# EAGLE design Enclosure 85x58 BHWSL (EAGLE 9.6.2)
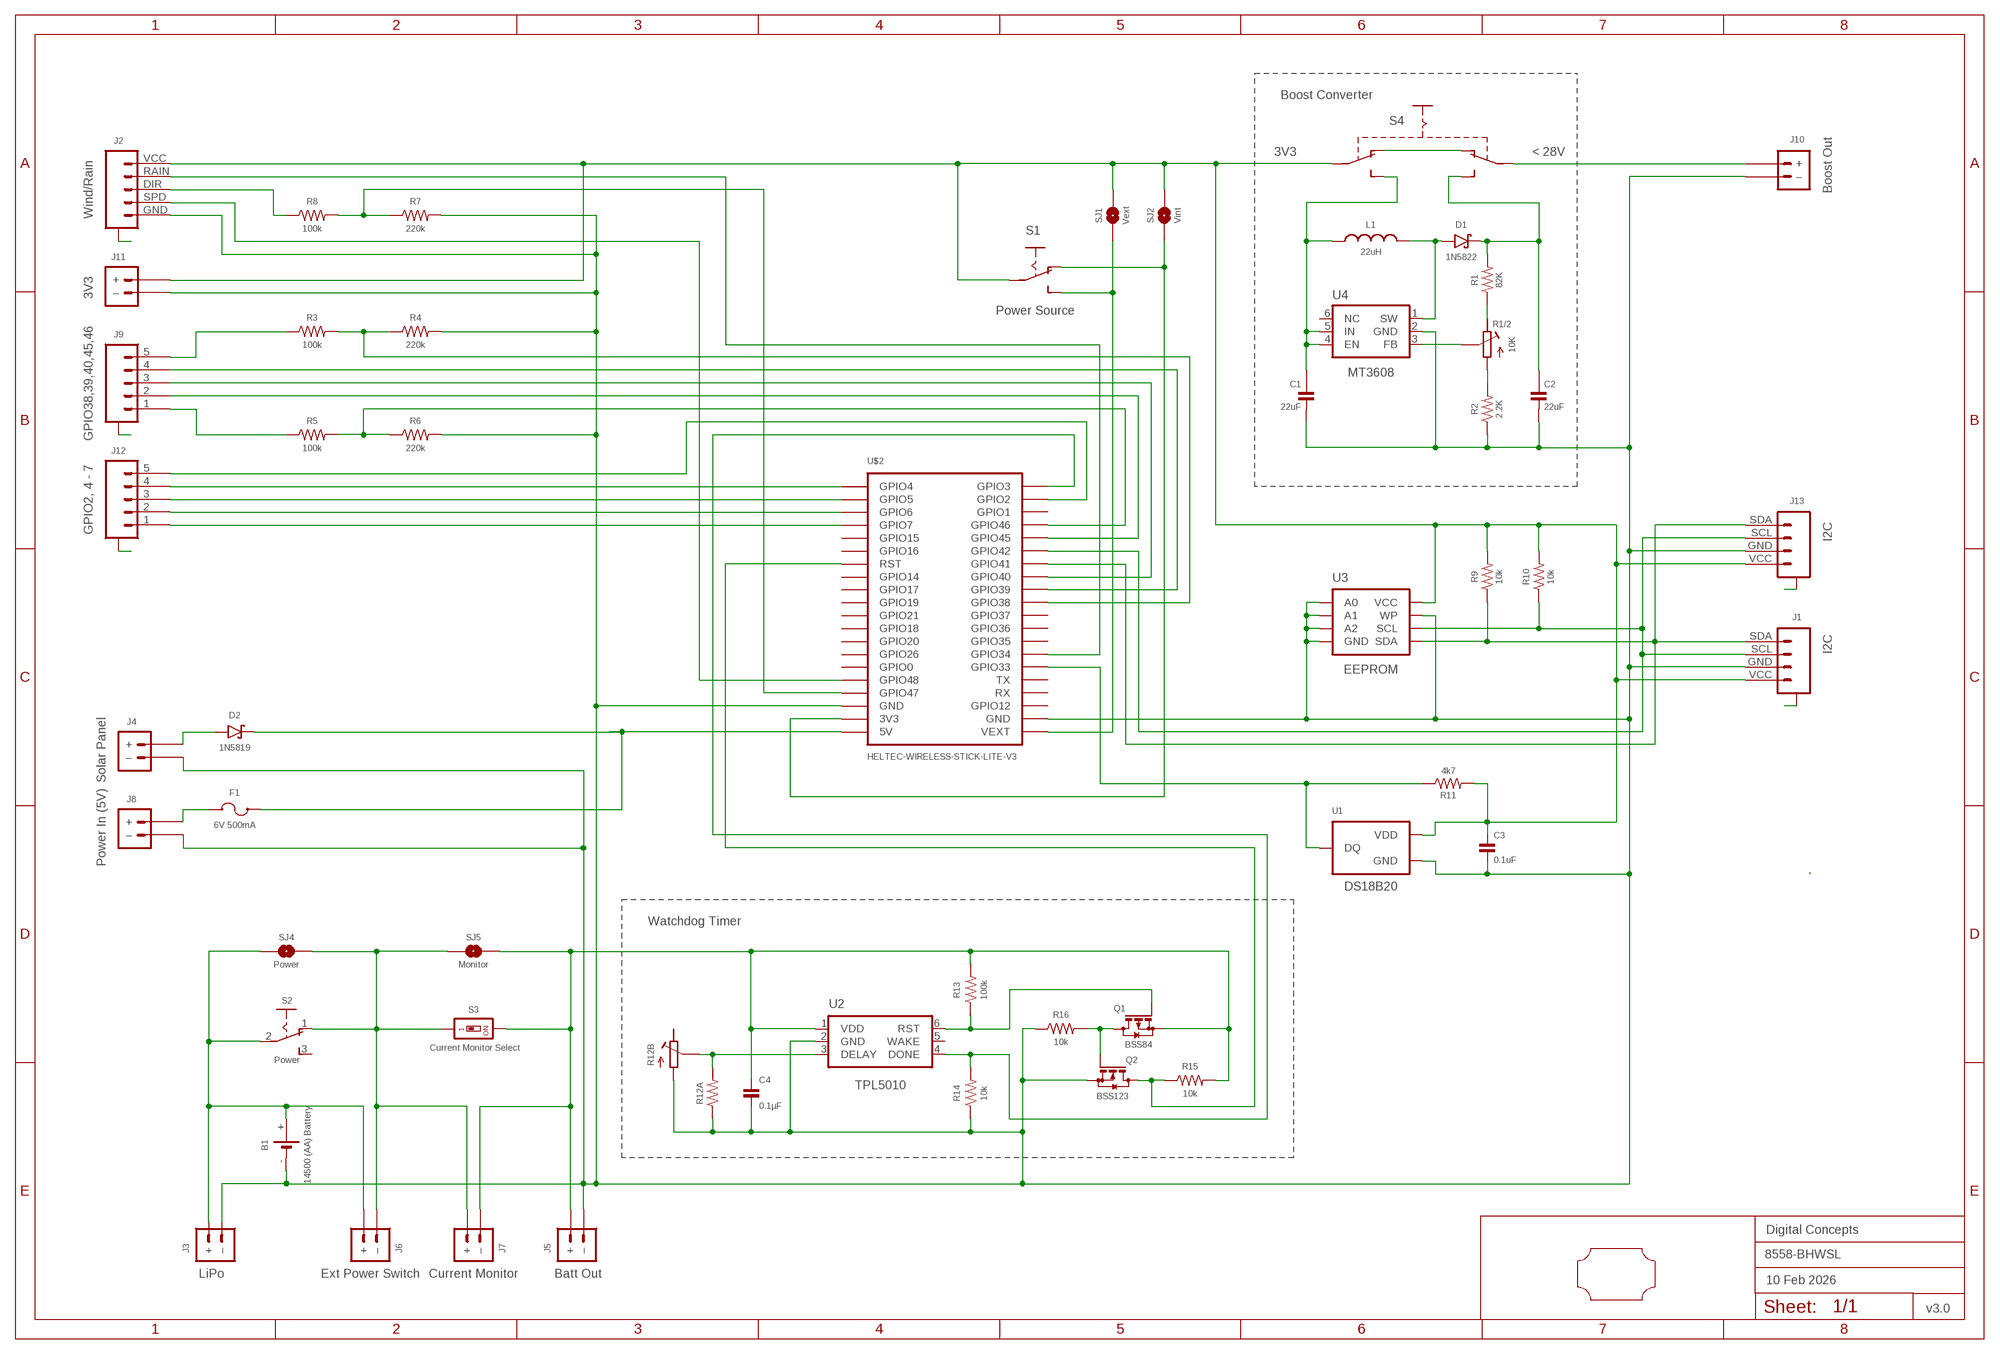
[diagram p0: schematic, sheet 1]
FRAME2 (A3L-LOC): DATE: 10 Feb 2026; OWNER: Digital Concepts; TITLE: 8558-BHWSL; VERSION: v3.0

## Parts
B1  14500 (AA) Battery  BATTERY-HOLDER-14500(AA)  [BATTERY-14500]
C1  22uF  CAPACITOR-1206  [C1206]
C2  22uF  CAPACITOR-1206  [C1206]
C3  0.1uF  CAPACITOR-0805  [C0805]
C4  0.1µF  CAPACITOR-0805  [C0805]
D1  1N5822  DIODE-SCHOTTKY-1N5822  [DIODE_SMB]
D2  1N5819  1N5819-SOD-123  [SOD-123]
F1  6V 500mA  MF-PSMF050X-2  [F0805]
J1  I2C  JST-SH1.0-4-SMD-VERTICAL-I2C  [JST-SH1.0-4-SMD-VERTICAL-I2C]
J2  Wind/Rain  JST-SH1.0-5-SMD-VERTICAL-WEATHER  [JST-SH1.0-5-SMD-VERTICAL-WEATHER]
J3  LiPo  JST-PH2.0-2-MALE-HORIZONTALJST-PTH-2  [JST-PH2.0-2-HORIZONTAL]
J4  Solar Panel  JST-PH2.0-2-VERTICAL-POWER  [JST-PH2.0-2-VERTICAL-POWER]
J5  Batt Out  JST-GH1.25-2-HORIZONTAL-POWER  [JST-GH1.25-2-HORIZONTAL]
J6  Ext Power Switch  JST-PH2.0-2-DUAL-POWERJST-PTH-2  [JST-PH2.0-2-DUAL-POWER]
J7  Current Monitor  JST-PH2.0-2-HORIZONTAL-POWERJST-PTH-2  [JST-PH2.0-2-HORIZONTAL-POWER@1]
J8  Power In (5V)  JST-PH2.0-2-H-POWER  [JST-PH2.0-2-HORIZONTAL-POWER]
J9  GPIO38,39,40,45,46  JST-SH1.0-5-SMD-HORIZONTAL  [JST-SH1.0-5-SMD-HORIZONTAL]
J10  Boost Out  JST-PH2.0-2-H-POWER  [JST-PH2.0-2-HORIZONTAL-POWER]
J11  3V3  JST-PH2.0-2-H-POWER  [JST-PH2.0-2-HORIZONTAL-POWER]
J12  GPIO2, 4 - 7  JST-SH1.0-5-SMD-HORIZONTAL  [JST-SH1.0-5-SMD-HORIZONTAL]
J13  I2C  JST-SH1.0-4-SMD-HORIZONTAL-I2C  [JST-SH1.0-4-SMD-HORIZONTAL-I2C]
L1  22uH  INDUCTOR-CDRH104R/6D28L5038P  [CDRH104R+6D28]
Q1  BSS84  MOSFET-BSS84  [SOT23-3]
Q2  BSS123  MOSFET-BSS123  [SOT23-3]
R1  82K  RESISTORR0805  [R0805]
R1/2  10K  RESISTOR-TRIMM-BAOTER-HORIZONTAL  [RTRIM64P]
R2  2.2K  RESISTORR0805  [R0805]
R3  100k  RESISTORR0805  [R0805]
R4  220k  RESISTORR0805  [R0805]
R5  100k  RESISTORR0805  [R0805]
R6  220k  RESISTORR0805  [R0805]
R7  220k  RESISTORR0805  [R0805]
R8  100k  RESISTORR0805  [R0805]
R9  10k  RESISTORR0805  [R0805]
R10  10k  RESISTORR0805  [R0805]
R11  4k7  RESISTORR0805  [R0805]
R12A  RESISTORR0805  [R0805]
R12B  RESISTOR-TRIMM-33  [RTRIM3*3]
R13  100k  RESISTORR0805  [R0805]
R14  10k  RESISTORR0805  [R0805]
R15  10k  RESISTORR0805  [R0805]
R16  10k  RESISTORR0805  [R0805]
S1  Power Source  SWITCH-SLIDE-SPDT-SMT  [SWITCH-SPDT-SMT]
S2  Power  SWITCH-SLIDE-SPDT  [SWITCH-SLIDE-SPDT]
S3  Current Monitor Select  SWITCH-DIP-SWS001  [SMD-001]
S4  SWITCH-SLIDE-DPDT-PTH-S  [SWITCH-DPDT-PTH]
SJ1  Vext  SJ  [SJ]
SJ2  Vint  SJ-V-1  [SJ-VIA-1]
SJ4  Power  SJ  [SJ]
SJ5  Monitor  SJ  [SJ]
U1  DS18B20  THERMOMETER-DS18B20  [TO-92]
U2  TPL5010  TPL5010DDCR  [SOT-23-6]
U3  EEPROM  AT24CXX-EEPROM  [SOP-8]
U4  MT3608  [SOT-23-6@1]
U$1  PCB-OUTLINE-85X58  [PROTO-28X18-OUTLINE]
U$2  HELTEC-WIRELESS-STICK-LITE-V3  [HELTEC-WIRELESS-STICK-LITE-V3]

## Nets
A1: J1.A@1(A) J1.A@4(A)
A2: J2.A@1(A) J2.A@5(A)
A9: J9.A@1(A) J9.A@5(A)
A12: J12.A@1(A) J12.A@5(A)
A13: J13.A@1(A) J13.A@4(A)
GND: B1.- C1.2 C2.2 C3.2 C4.2 J1.GND J2.GND J3.-(–) J4.-(–) J5.-(–) J8.-(–) J10.-(–) J11.-(–) J13.GND Q2.2(S) R2.1 R4.2 R6.2 R7.2 R12A.1 R12B.1(A) R14.1 R16.1 U1.1(GND) U2.2(GND) U3.P$1(A0) U3.P$2(A1) U3.P$3(A2) U3.P$4(GND) U3.P$7(WP) U4.2(GND) U$2.GND@18(GND) U$2.GND@22(GND)
N$1: D2.A J4.+
N$2: J2.DIR R8.1
N$3: R1.1 R1/2.3(E)
N$4: B1.+ J3.+ J6.+ S2.2(P) SJ4.2
N$5: D2.C F1.2 U$2.5V
N$6: D1.A L1.1 U4.1(SW)
N$7: R7.1 R8.2 U$2.GPIO47
N$8: J1.SCL J13.SCL R10.1 U3.P$6(SCL) U$2.GPIO42
N$9: J9.1 R5.1
N$10: J12.5 U$2.GPIO2
N$11: J1.SDA J13.SDA R9.1 U3.P$5(SDA) U$2.GPIO41
N$12: J2.SPD U$2.GPIO48
N$13: S1.P$1(O) SJ2.2 U$2.3V3
N$14: C4.1 J5.+ J7.-(–) Q1.2(S) R13.2 R15.2 S3.2 SJ5.1 U2.1(VDD)
N$15: J12.4 U$2.GPIO4
N$16: J12.3 U$2.GPIO5
N$18: R11.1 U1.2(DQ) U$2.GPIO33
N$19: J12.2 U$2.GPIO6
N$20: C2.1 D1.C R1.2 S4.P$3(S1)
N$21: S1.P$2(S) SJ1.2 U$2.VEXT
N$22: J2.RAIN U$2.GPIO34
N$23: R1/2.1(A) R2.2
N$24: R1/2.2(S) U4.3(FB)
N$25: C1.1 L1.2 S4.P$6(S2) U4.4(EN) U4.5(IN)
N$26: S4.P$1(O1) S4.P$4(O2)
N$27: J10.+ S4.P$2(P1)
N$28: J12.1 U$2.GPIO7
N$29: J9.2 U$2.GPIO45
N$30: J9.3 U$2.GPIO40
N$31: J9.4 U$2.GPIO39
N$32: J9.5 R3.1
N$33: R3.2 R4.1 U$2.GPIO38
N$34: R5.2 R6.1 U$2.GPIO46
N$35: Q2.3(D) R15.1 U$2.RST
N$38: R14.2 U2.4(DONE) U$2.GPIO3
N$39: J6.-(–) J7.+ S2.1(O) S3.1 SJ4.1 SJ5.2
N$40: F1.1 J8.+
N$43: Q1.3(D) Q2.1(G) R16.2
N$44: Q1.1(G) R13.1 U2.6(RST)
N$46: R12A.2 R12B.2(S) U2.3(DELAY)
VCC: C3.1 J1.VCC J2.VCC J11.+ J13.VCC R9.2 R10.2 R11.2 S1.COMMON(P) S4.P$5(P2) SJ1.1 SJ2.1 SJ2.1@V U1.3(VDD) U3.P$8(VCC)
Unconnected: R12B.3(E) S2.3(S) U2.5(WAKE) U4.6(NC) U$2.GPIO0 U$2.GPIO1 U$2.GPIO12 U$2.GPIO14 U$2.GPIO15 U$2.GPIO16 U$2.GPIO17 U$2.GPIO18 U$2.GPIO19 U$2.GPIO20 U$2.GPIO21 U$2.GPIO26 U$2.GPIO35 U$2.GPIO36 U$2.GPIO37 U$2.RX U$2.TX

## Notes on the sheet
- Boost Converter
- 3V3 | < 28V
- Watchdog Timer

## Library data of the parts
B1 = digitalconcepts:BATTERY-HOLDER-14500(AA): 14500 (AA) battery holder
C1 C2 = digitalconcepts:CAPACITOR-1206: 1206 Capacitor
C3 C4 = digitalconcepts:CAPACITOR-0805: 0805 Capacitor
D1 = digitalconcepts:DIODE-SCHOTTKY-1N5822: 1N5822 Schottky Diode SMB
D2 = digitalconcepts:1N5819-SOD-123: 1N5819 Schottky Diode SOD-123
F1 = digitalconcepts:MF-PSMF050X-2: PTC Resettable Fuse
J1 = digitalconcepts:JST-SH1.0-4-SMD-VERTICAL-I2C: JST SH1.0 4P SMD I2C vertical connector
J2 = digitalconcepts:JST-SH1.0-5-SMD-VERTICAL-WEATHER: JST SH1.0 5P SMD Vertical Weather Connector
J3 = digitalconcepts:JST-PH2.0-2-MALE-HORIZONTAL: PH2.0 2P Right Angle PCB Connector; PROD_ID: CONN-09863; SKU: PRT-09914
J4 = digitalconcepts:JST-PH2.0-2-VERTICAL-POWER: JST PH2.0 2P PTH Connector (Power)
J5 = digitalconcepts:JST-GH1.25-2-HORIZONTAL-POWER: JST GH1.25 2P PTH Connector (Power)
J6 = digitalconcepts:JST-PH2.0-2-DUAL-POWER: JST PH2.0 2P PTH Dual-Side Connector (Power); PROD_ID: CONN-09863; SKU: PRT-09914
J7 = digitalconcepts:JST-PH2.0-2-HORIZONTAL-POWER: PH2.0 2P Right Angle PCB Connector; PROD_ID: CONN-09863; SKU: PRT-09914
J8 J10 J11 = digitalconcepts:JST-PH2.0-2-H-POWER: JST PH2.0 2P Right Angle Connector with power pin labelling
J9 J12 = digitalconcepts:JST-SH1.0-5-SMD-HORIZONTAL: JST SH1.0 5P SMD horizontal connector
J13 = digitalconcepts:JST-SH1.0-4-SMD-HORIZONTAL-I2C: JST SH1.0 4P SMD I2C horizontal connector
L1 = digitalconcepts:INDUCTOR-CDRH104R/6D28: Inductor; SPICEPREFIX: L
Q1 = digitalconcepts:MOSFET-BSS84: P-CHANNEL MOS FET
Q2 = digitalconcepts:MOSFET-BSS123: N-CHANNEL MOS FET
R1-R11 R12A R13-R16 = digitalconcepts:RESISTOR: Resistor; SPICEPREFIX: R
R1/2 = digitalconcepts:RESISTOR-TRIMM-BAOTER-HORIZONTAL: Trimm Resistor - Horizontal BAOTER
R12B = digitalconcepts:RESISTOR-TRIMM-3*3: Trimm Resistor - 3*3 SMD
S1 = digitalconcepts:SWITCH-SLIDE-SPDT-SMT: Mini Sliding Switch SPDT SMT
S2 = digitalconcepts:SWITCH-SLIDE-SPDT: Mini Sliding Switch SPDT
S3 = digitalconcepts:SWITCH-DIP-SWS001: SMD Dip Switch 1 pol.
S4 = digitalconcepts:SWITCH-SLIDE-DPDT-PTH-S: Switch DPDT PTH-S
SJ1 SJ4 SJ5 = digitalconcepts:SJ: Solder Jumper
SJ2 = digitalconcepts:SJ-V-1: Solder Jumper with single Pad Via
U1 = digitalconcepts:THERMOMETER-DS18B20: Digital Thermometer -55C-125C TO92-3; AVAILABILITY: Bad; DESCRIPTION: Temperature Sensor Digital, Local -55°C ~ 125°C 12 b 8-uMAX; MF: Maxim Integrated; MP: DS18B20; PACKAGE: TO-92 Maxim Integrated; PRICE: None
U2 = digitalconcepts:TPL5010DDCR: TPL5010 Nano-Power System Timer with Watchdog
U3 = digitalconcepts:AT24CXX-EEPROM: AT24Cxx EEPROM SOP-8
U4 = digitalconcepts:MT3608: MT3608 DC-DC Step-Up Voltage Converter
U$1 = digitalconcepts:PCB-OUTLINE-85X58: PCB outline for 85 x 58 enclosure
U$2 = digitalconcepts:HELTEC-WIRELESS-STICK-LITE-V3: Heltec Wireless Stick Lite V3 MCU

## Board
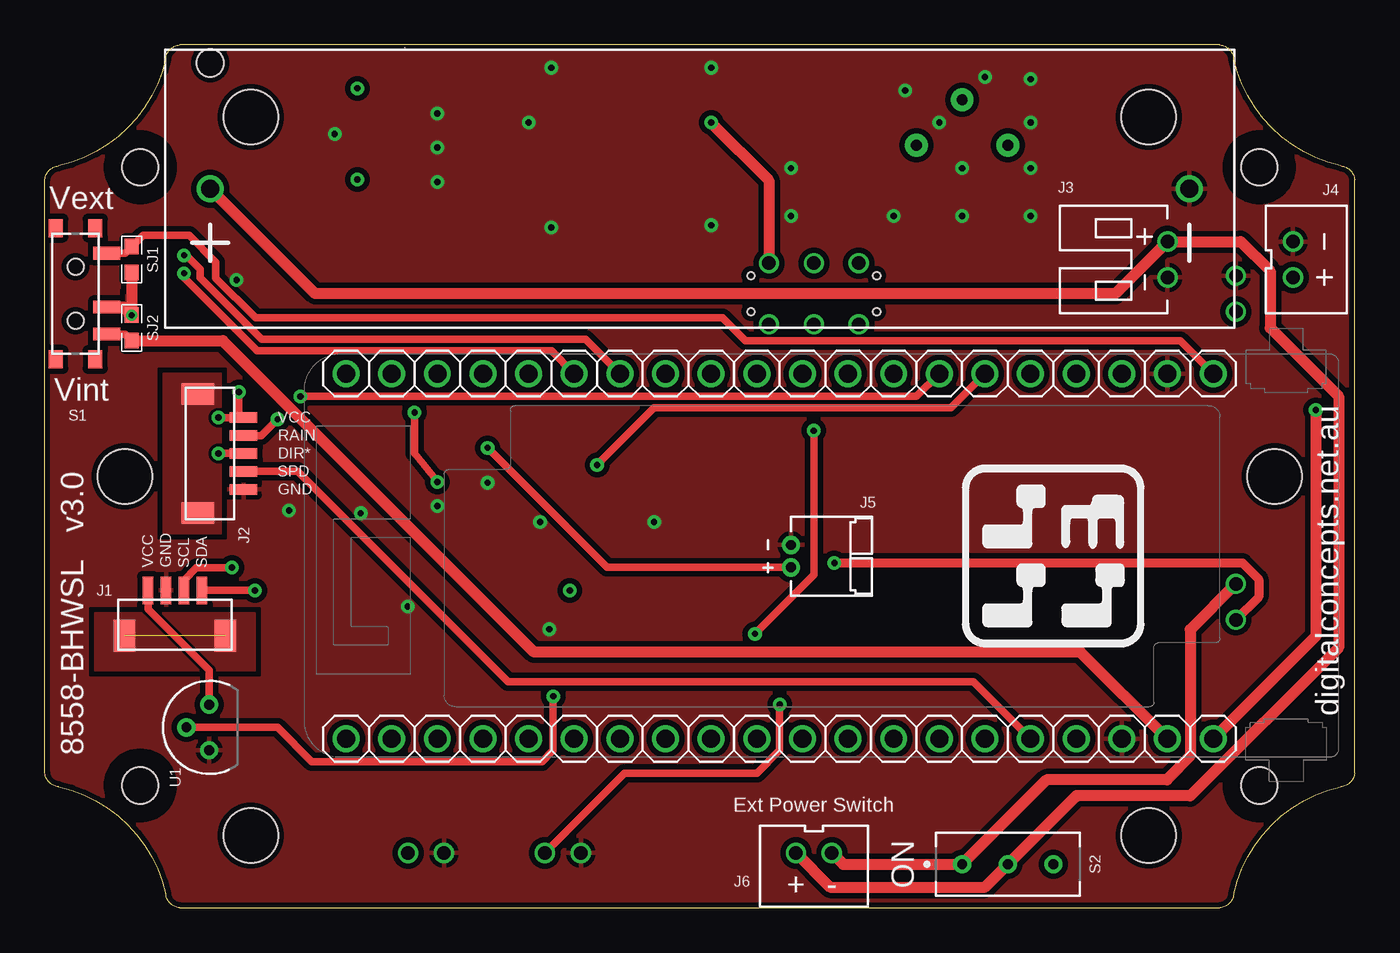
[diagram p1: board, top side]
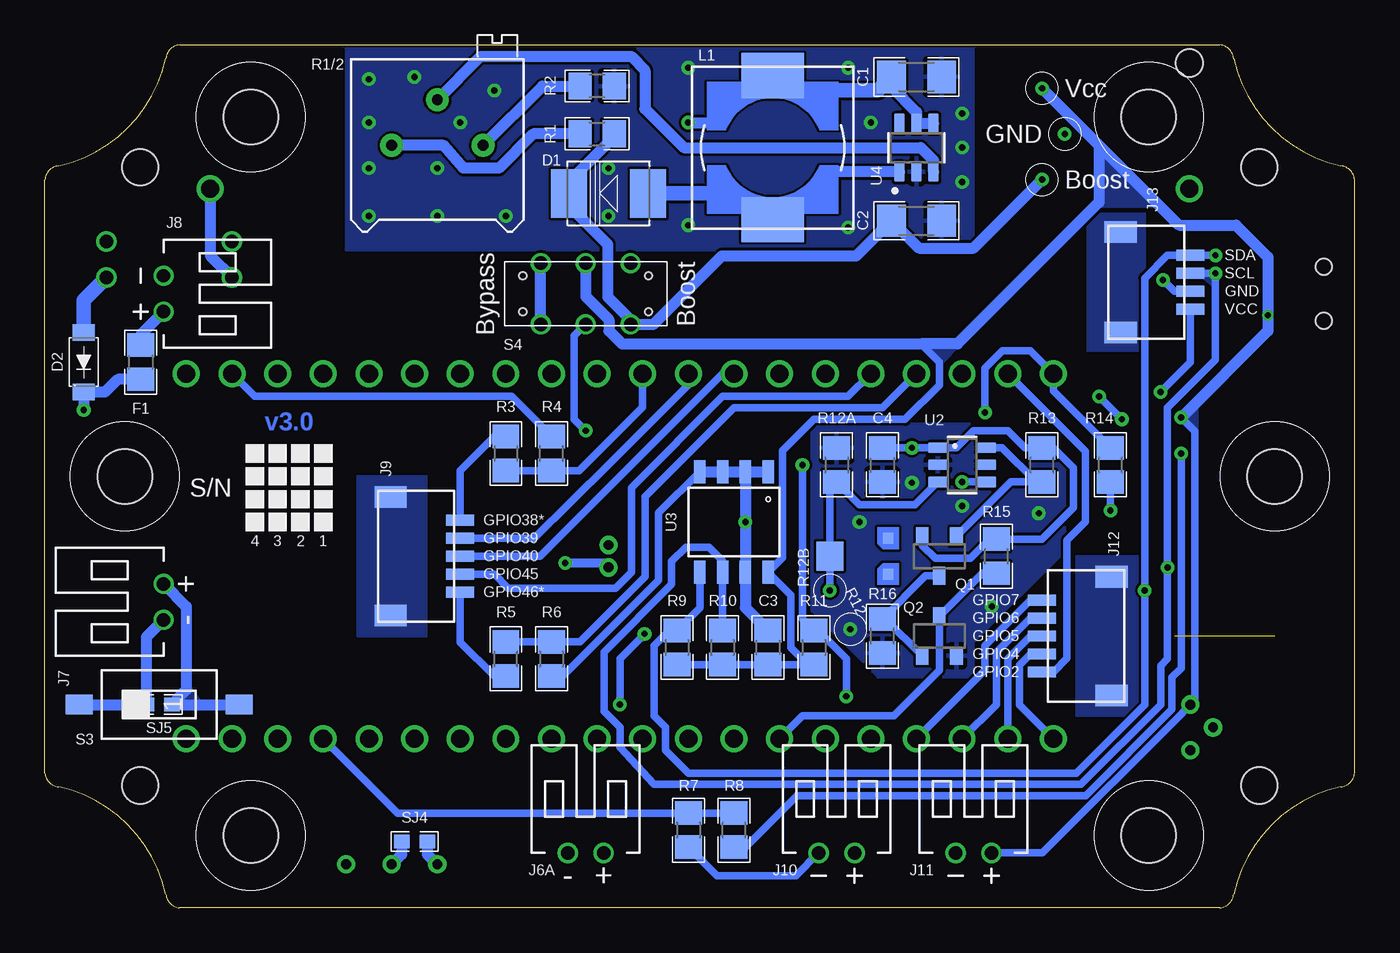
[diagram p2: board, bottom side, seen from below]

Size 72.9 x 48.01 mm. Coordinates in mm from the lower left corner, seen from the top.
Copper layers (1*16): Top 0.035mm / dielectric 1.5mm / Bottom 0.035mm
Design rules "default *": minimum track width 6mil, minimum drill 0.35mm, track to track 6mil, track to pad 6mil, pad to pad 6mil, via to via 6mil, smd to smd 6mil, copper to edge 6mil, drill to drill 6mil, minimum pad ring 1mil, minimum via ring 8mil, stop-mask expansion 4mil, vias tented up to drill 0mil, thermal gap 10mil

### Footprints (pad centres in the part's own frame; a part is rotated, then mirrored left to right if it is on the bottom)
BATTERY-14500 = drill 1: + -27.25,0; - 27.25,0 | hole 1.524: -27.25,7
C1206 = smd 1.6 x 1.8: 1 -1.4,0; 2 1.4,0
C0805 = smd 1.3 x 1.5: 1 -0.95,0; 2 0.95,0
DIODE_SMB = smd 2 x 2.7: A 2.2,0; C -2.2,0
SOD-123 = smd 0.91 x 1.22: A -1.65,0; C 1.65,0
F0805 = smd 1.3 x 1.5: 1 -0.95,0; 2 0.95,0
JST-SH1.0-4-SMD-VERTICAL-I2C = smd 1.2 x 1.8: A@1 2.8,-0.015; A@4 -2.8,-0.015 | smd 0.6 x 1.55: GND 0.5,-2.54; SCL -0.5,-2.54; SDA -1.5,-2.54; VCC 1.5,-2.54
JST-SH1.0-5-SMD-VERTICAL-WEATHER = smd 1.2 x 1.8: A@1 3.3,-0.015; A@5 -3.3,-0.015 | smd 0.6 x 1.55: DIR 0,-2.54; GND -2,-2.54; RAIN 1,-2.54; SPD -1,-2.54; VCC 2,-2.54
JST-PH2.0-2-HORIZONTAL = drill 0.75: + 1,0; - -1,0
JST-PH2.0-2-VERTICAL-POWER = drill 0.75: + -1,0; - 1,0
JST-GH1.25-2-HORIZONTAL = drill 0.55 pad 1.016: + -0.625,0; - 0.625,0
JST-PH2.0-2-DUAL-POWER = drill 0.75: + 1,0; - -1,0
JST-PH2.0-2-HORIZONTAL-POWER@1 = drill 0.75: + 1,0; - -1,0
JST-PH2.0-2-HORIZONTAL-POWER = drill 0.75: + 1,0; - -1,0
JST-SH1.0-5-SMD-HORIZONTAL = smd 0.6 x 1.55: 1 2,2.54; 2 1,2.54; 3 0,2.54; 4 -1,2.54; 5 -2,2.54 | smd 1.2 x 1.8: A@1 3.3,-1.335; A@5 -3.3,-1.335
JST-SH1.0-4-SMD-HORIZONTAL-I2C = smd 1.2 x 1.8: A@1 2.8,-1.335; A@4 -2.8,-1.335 | smd 0.6 x 1.55: GND 0.5,2.54; SCL -0.5,2.54; SDA -1.5,2.54; VCC 1.5,2.54
CDRH104R+6D28 = smd 2.5 x 3.5: 1 -4,0; 2 4,0
SOT23-3 = smd 0.7 x 1: 1 -0.95,-1.1; 2 0.95,-1.1; 3 0,1.1
R0805 = smd 1.3 x 1.5: 1 -0.95,0; 2 0.95,0
RTRIM64P = drill 0.61 pad 1.27: 1 0,-2.54; 2 2.54,0; 3 0,2.54
RTRIM3*3 = smd 0.6 x 0.6: 1 -1,-1.6; 3 1,-1.6 | smd 1.6 x 1.5: 2 0,1.65
SWITCH-SPDT-SMT = smd 0.7 x 1.5: COMMON 0.75,1.75; P$1 2.25,1.75; P$2 -2.25,1.75 | smd 1 x 0.8: GND@1 3.65,-1.1; GND@2 3.65,1.1; GND@3 -3.65,1.1; GND@4 -3.65,-1.1 | hole 0.9: -1.5,0; 1.5,0
SWITCH-SLIDE-SPDT = drill 0.55 pad 1.016: 1 -2.54,0; 2 0,0; 3 2.54,0
SMD-001 = smd 1.1 x 1.5: 1 0,-4.45; 2 0,4.45
SWITCH-DPDT-PTH = drill 0.75: P$1 -1.7,2.5; P$2 -1.7,0; P$3 -1.7,-2.5; P$4 1.7,2.5; P$5 1.7,0; P$6 1.7,-2.5 | hole 0.42: 1,3.5; -1,3.5; 1,-3.5; -1,-3.5
SJ = smd 0.864 x 0.762: 1 -0.711,0; 2 0.711,0
SJ-VIA-1 = smd 0.864 x 0.762: 1 -0.711,0; 2 0.711,0 | drill 0.35 pad 0.61: 1@V -0.711,0
TO-92 = drill 0.55 pad 1.016: 1 -1.27,0; 2 0,1.27; 3 1.27,0
SOT-23-6 = smd 1.1 x 0.6: 1 -1.35,0.95; 2 -1.35,0; 3 -1.35,-0.95; 4 1.35,-0.95; 5 1.35,0; 6 1.35,0.95
SOP-8 = smd 0.635 x 1.27: P$1 -1.905,-2.794; P$2 -0.635,-2.794; P$3 0.635,-2.794; P$4 1.905,-2.794; P$5 1.905,2.794; P$6 0.635,2.794; P$7 -0.635,2.794; P$8 -1.905,2.794
SOT-23-6@1 = smd 1.1 x 0.6: 1 -1.35,0.95; 2 -1.35,0; 3 -1.35,-0.95; 4 1.35,-0.95; 5 1.35,0; 6 1.35,0.95
PROTO-28X18-OUTLINE = hole 2.032: -31.14,17.196; -31.14,-17.196; 31.14,-17.196; 31.14,17.196 | hole 3.048: -24.994,19.99; -32.004,0; -24.994,-19.99; 24.994,-19.99; 32.004,0; 24.994,19.99
HELTEC-WIRELESS-STICK-LITE-V3 = drill 1: 3V3 0,45.72; 5V 0,48.26; GND@18 0,43.18; GND@22 -20.32,45.72; GPIO0 0,35.56; GPIO1 -20.32,5.08; GPIO2 -20.32,2.54; GPIO3 -20.32,0; GPIO4 0,0; GPIO5 0,2.54; GPIO6 0,5.08; GPIO7 0,7.62; GPIO12 -20.32,43.18; GPIO14 0,17.78; GPIO15 0,10.16; GPIO16 0,12.7; GPIO17 0,20.32; GPIO18 0,27.94; GPIO19 0,22.86; GPIO20 0,30.48; GPIO21 0,25.4; GPIO26 0,33.02; GPIO33 -20.32,35.56; GPIO34 -20.32,33.02; GPIO35 -20.32,30.48; GPIO36 -20.32,27.94; GPIO37 -20.32,25.4; GPIO38 -20.32,22.86; GPIO39 -20.32,20.32; GPIO40 -20.32,17.78; GPIO41 -20.32,15.24; GPIO42 -20.32,12.7; GPIO45 -20.32,10.16; GPIO46 -20.32,7.62; GPIO47 0,40.64; GPIO48 0,38.1; RST 0,15.24; RX -20.32,40.64; TX -20.32,38.1; VEXT -20.32,48.26

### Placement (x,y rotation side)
B1  36.45,40.01 0 top
C1  24.38,46.23 0 bottom
C2  24.38,38.23 0 bottom
C3  32.64,14.48 90 bottom
C4  26.29,24.64 270 bottom
D1  41.53,39.75 0 bottom
D2  70.74,30.35 270 bottom
F1  67.56,30.35 270 bottom
J1  7.24,15.11 180 top
J2  8.51,25.27 90 top
J3  62.48,36.07 90 top
J4  69.47,36.07 90 top
J5  41.53,19.56 90 top
J6  42.8,3.05 0 bottom
J7  66.29,17.02 90 bottom
J8  66.29,34.16 270 bottom
J9  52.32,19.56 270 bottom
J10  28.83,3.05 0 bottom
J11  21.21,3.05 0 bottom
J12  14.86,15.11 90 bottom
J13  11.68,34.8 270 bottom
L1  32.38,42.29 90 bottom
Q1  23.11,19.56 180 bottom
Q2  23.11,15.11 0 bottom
R1  42.16,43.05 0 bottom
R1/2  51.05,42.42 90 bottom
R2  42.16,45.72 180 bottom
R3  47.24,25.27 270 bottom
R4  44.7,25.27 90 bottom
R5  47.24,13.84 90 bottom
R6  44.7,13.84 270 bottom
R7  37.08,4.32 270 bottom
R8  34.54,4.32 90 bottom
R9  37.72,14.48 270 bottom
R10  35.18,14.48 270 bottom
R11  30.1,14.48 270 bottom
R12A  28.83,24.64 270 bottom
R12B  27.56,19.56 90 bottom
R13  17.4,24.64 90 bottom
R14  13.59,24.64 90 bottom
R15  19.94,19.56 90 bottom
R16  26.29,15.11 90 bottom
S1  1.7,34.16 270 top
S2  53.59,2.41 0 top
S3  66.55,11.3 90 bottom
S4  42.8,34.16 90 bottom
SJ1  4.83,36.07 90 top
SJ2  4.83,32.26 270 top
SJ4  52.32,3.68 180 bottom
SJ5  66.55,11.3 0 bottom
U1  9.14,10.03 90 top
U2  21.84,24.64 0 bottom
U3  34.54,21.46 180 bottom
U4  24.38,42.29 90 bottom
U$1  36.45,24 0 top
U$2  16.76,9.4 270 top

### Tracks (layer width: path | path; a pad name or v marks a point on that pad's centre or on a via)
$X1
  cutout Bottom: 67.59,43.23 arc180 67.59,39.17 arc180
$X2
  cutout Bottom: 67.59,8.84 arc180 67.59,4.78 arc180
$X3
  cutout Bottom: 5.31,8.84 arc180 5.31,4.78 arc180
$X4
  cutout Bottom: 5.31,43.23 arc180 5.31,39.17 arc180
$X5
  cutout Top: 5.31,43.23 arc180 5.31,39.17 arc180
$X6
  cutout Top: 67.59,43.23 arc180 67.59,39.17 arc180
$X7
  cutout Top: 67.59,8.84 arc180 67.59,4.78 arc180
$X8
  cutout Top: 5.31,8.84 arc180 5.31,4.78 arc180
A1  (1 unrouted)
  pour Top (no thermals): 11.68,16.38 2.79,16.38 2.79,13.21 11.68,13.21
A2
  pour Top (no thermals): 6.6,29.72 9.78,29.72 9.78,20.83 6.6,20.83
A9
  pour Bottom (no thermals): 55.5,24 51.69,24 51.69,15.11 55.5,15.11
A12
  pour Bottom (no thermals): 15.49,19.56 11.68,19.56 11.68,10.67 15.49,10.67
A13
  pour Bottom (no thermals): 14.86,38.61 11.68,38.61 11.68,30.99 14.86,30.99
GND  (via drill 0.35)
  Bottom 0.406: J10.- 31.1,1.78 35.49,1.78 R7.2 | U$2.GND@22 61.21,28.45 46.93,28.45 R4.2 | R6.2 44.07,12.89 38.73,18.23 38.73,21.97 U3.P$4 | v10.67,34.93 10.03,34.3 J13.GND | v13.59,22.1 R14.1
  Bottom 0.61: U3.P$4 U3.P$3 U3.P$2 | U3.P$2 U3.P$1 | B1.- 63.7,36.28 J3.- | C3.2 33.91,16.7 U3.P$7 v33.91,21.46 U3.P$2
  other vias: 21.84,44.2 26.92,43.69 37.08,37.97 37.08,46.74 47.88,45.47 52.32,46.23 41.53,38.48 47.24,38.48 51.05,38.48 51.05,41.15 54.86,38.48 54.86,41.15 54.86,46.1 21.84,40.39 49.78,43.69 54.86,43.69 28.19,37.85 41.53,41.15 16.13,43.05 21.84,42.29 28.19,46.74 21.84,22.35 24.64,23.65 20.19,16.76 27.56,21.46 28.07,15.49 17.58,21.95
  pour Top (isolate 0.305, rank 2): -2.08,49.93 -2.08,-1.97 74.92,-1.97 74.92,49.93
  pour Bottom (rank 2): 21.21,48.13 21.21,36.58 56.13,36.58 56.13,48.13
  pour Bottom: 30.23,26.92 16.13,26.92 16.13,19.81 21.21,14.73 21.21,12.83 26.54,12.83 30.23,16.51
N$1
  Bottom 0.813: D2.A 70.74,33.8 J4.+
N$2  (via drill 0.35)
  Top 0.406: v9.65,25.27 J2.DIR
  Bottom 0.406: R8.1 33.91,3.37 31.04,6.24 14.97,6.24 10.16,11.05 10.16,12.83 9.65,13.34 v9.65,25.27
N$3
  Bottom 0.61: R1.1 45.72,43.05 47.62,41.15 49.6,41.15 50.69,42.42 R1/2.3
N$4
  Top 0.61: B1.+ 15.04,34.16 59.58,34.16 J3.+ 66.56,37.07 68.2,35.43 68.2,32.26 72.01,28.45 72.01,14.48 63.75,6.22 57.48,6.22 | 57.48,6.22 57.42,6.24 S2.2 52.32,1.14 43.7,1.14 J6.+ | 57.48,6.22
  Bottom 0.61: SJ4.2 53.03,2.97 S2.2
N$5  (via drill 0.35)
  Top 0.61: U$2.5V 70.74,15.11 v70.74,27.69
  Bottom 0.61: v70.74,27.69 D2.C 69.55,28.7 68.84,29.4 F1.2
N$6
  Bottom 0.61: L1.1 31.75,38.29 29.1,40.94 U4.1
  Bottom 0.813: D1.A 34.54,39.75 33.08,38.29 L1.1
N$7
  Bottom 0.406: U$2.GPIO47 53.27,5.27 R7.1 R8.2
N$8  (via drill 0.35)
  Top 0.406: J1.SCL 7.74,18.23 8.43,18.92 v10.41,18.92 | U$2.GPIO42 28.19,30.99 11.81,30.99 7.75,35.05 v7.75,35.3
  Bottom 0.406: R10.1 U3.P$6 35.18,19.3 35.94,20.07 37.21,20.07 38.01,19.27 38.01,18 41.78,14.22 41.78,10.92 40.89,10.03 40.89,8.93 38.99,6.86 15.24,6.86 10.79,11.3 10.79,13.46 10.41,13.84 v10.41,18.92 10.41,27.81 7.75,30.48 v7.75,35.3 J13.SCL
  pour Bottom (no thermals): 8.51,35.3 7.75,35.3 7.75,34.66
N$9
  Bottom 0.406: J9.1 49.78,14.77 47.91,12.89 R5.1
N$10
  Bottom 0.406: J12.5 16.76,13.11 16,13.88 16,20.45 14.99,21.46 14.99,25.4 U$2.GPIO2
N$11  (via drill 0.35)
  Top 0.406: J1.SDA v11.68,17.65 | U$2.GPIO41 30.1,31.62 12.06,31.62 8.64,35.05 8.64,35.54 7.87,36.3 v7.75,36.3
  Bottom 0.406: U3.P$5 36.45,16.7 R9.1 38.12,15.43 38.99,14.56 38.99,10.67 38.35,10.03 38.35,8.76 37.08,7.49 15.49,7.49 11.68,11.3 v11.68,17.65 11.68,35.03 10.41,36.3 J13.SDA v7.75,36.3
N$12
  Top 0.406: U$2.GPIO48 51.69,12.57 25.78,12.57 14.29,24.07 14.08,24.27 J2.SPD
N$13
  Top 0.406: SJ2.2 4.46,31.91 S1.P$1
  Top 0.61: SJ2.2 9.91,31.55 27.23,14.22 57.64,14.22 U$2.3V3
N$14  (via drill 0.35)
  Top 0.406: J5.+ 31.29,18.93 v24.64,25.59
  Top 0.508: v43.94,19.18 66.67,19.18 67.56,18.29 67.56,17.29 J7.-
  Bottom 0.406: Q1.2 24.06,20.15 23.34,19.43 21.4,19.43 20.32,20.51 R15.2 17.4,20.51 15.65,22.26 15.65,24.48 16.76,25.59 R13.2 18.35,25.59 19.3,26.54 21.21,26.54 22.16,25.59 U2.1 v24.64,25.59 C4.1
  Bottom 0.508: J5.+ 41.77,19.18 v43.94,19.18
  Bottom 0.61: S3.2 SJ5.1 67.26,15.05 J7.-
N$15
  Bottom 0.406: J12.4 18.03,14.11 18.67,13.48 18.67,11.3 U$2.GPIO4
N$16
  Bottom 0.406: J12.3 18.03,15.11 19.3,13.84 U$2.GPIO5
N$18  (via drill 0.35)
  Top 0.406: U$2.GPIO33 50.42,27.81 33.91,27.81 v30.73,24.64 | v28.29,11.76 28.29,8.76 27.66,8.13 14.86,8.13 12.95,10.03 U1.2
  Bottom 0.406: v30.73,24.64 30.73,16.06 R11.1 29.88,15.43 28.29,13.84 v28.29,11.76
N$19
  Bottom 0.406: J12.2 18.03,16.11 19.94,14.21 19.94,11.3 U$2.GPIO6
N$20  (via drill 0.35)
  Bottom 0.61: v17.4,40.51 21.21,36.7 24.26,36.7 C2.1 27.74,36.27 35.22,36.27 39.03,32.46 S4.P$3 40.3,32.72 41.57,33.99 41.57,36.91 43.73,39.07 D1.C 43.73,40.39 41.21,42.91 R1.2
N$21
  Top 0.406: S1.P$2 4.46,36.41 SJ1.2 5.46,37.41 8.02,37.41 9.51,35.93 9.51,35.04 11.72,32.82 37.72,32.82 38.99,31.55 63.2,31.55 U$2.VEXT
N$22  (via drill 0.35)
  Top 0.406: U$2.GPIO34 48.51,28.45 v14.22,28.45 | v12.95,27.18 12.05,26.27 J2.RAIN
  Bottom 0.406: v14.22,28.45 v12.95,27.18
N$23
  Bottom 0.61: R1/2.1 45.21,45.72 R2.2
N$24
  Bottom 0.61: R1/2.2 48.64,47.37 40.26,47.37 39.5,46.61 39.5,44.45 37.34,42.29 24.15,42.29 23.43,41.58 U4.3
N$25  (via drill 0.35)
  Top 0.61: v37.08,43.69 40.3,40.47 S4.P$6
  Bottom 0.61: C1.1 25.78,45.67 24.38,44.27 U4.5 U4.4 | v37.08,43.69 35.81,43.69 33.21,46.29 L1.2
  Bottom 0.813: C1.1 26.53,45.48 31.58,45.48 L1.2
N$26
  Bottom 0.61: S4.P$1 S4.P$4
N$27  (via drill 0.35)
  Top 0.406: J10.+ 32.27,7.49 39.62,7.49 40.89,8.76 v40.89,11.3 | v39.52,15.24 42.8,18.52 v42.8,26.54
  Bottom 0.406: v40.89,11.3 40.89,13.84 39.52,15.22 v39.52,15.24 | v42.8,26.54 43.43,27.18 43.43,31.83 S4.P$2
N$28
  Bottom 0.406: J12.1 18.03,17.11 20.57,14.57 20.57,13.21 U$2.GPIO7
N$29
  Bottom 0.406: J9.2 47.88,18.56 47.11,17.79 41.14,17.79 40.26,18.67 40.26,23.37 35.18,28.45 28.19,28.45 U$2.GPIO45
N$30
  Bottom 0.406: J9.3 45.34,19.56 35.18,29.72 U$2.GPIO40
N$31
  Bottom 0.406: U$2.GPIO39 37.08,29.11 41.53,24.64 45.67,20.56 J9.4
N$32
  Bottom 0.406: J9.5 49.78,24.32 47.88,26.22 R3.1
N$33
  Bottom 0.406: U$2.GPIO38 39.62,27.85 43.15,24.32 R4.1 R3.2
N$34
  Bottom 0.406: R5.2 R6.1 43.12,14.79 39.5,18.41 39.5,22.86 34.54,27.81 26.29,27.81 U$2.GPIO46
N$35
  Bottom 0.406: R15.1 20.72,18.61 Q2.3 23.11,13.21 25.65,10.67 30.73,10.67 U$2.RST
N$38  (via drill 0.35)
  Top 0.406: v20.57,27.56 20.57,25.27 v21.84,23.69
  Bottom 0.406: U2.4 v21.84,23.69 | v20.57,27.56 20.57,30.01 19.6,30.99 18.03,30.99 U$2.GPIO3 16.76,28.76 R14.2
N$39
  Top 0.61: J7.+ 63.75,15.48 63.75,8.46 62.46,7.11 55.75,7.11 S2.1 44.43,2.41 J6.-
  Bottom 0.61: J7.+ 65.02,16.75 65.02,12.12 SJ5.2 S3.1 | SJ4.1 51.61,2.97 S2.1
  pour Bottom: 65.85,11.3 65.02,12.12 64.39,11.3
N$40
  Bottom 0.61: J8.+ 67.56,31.89 F1.1
N$43
  Bottom 0.406: Q1.3 23.89,18.46 R16.2 26.11,16.06 Q2.1
N$44
  Bottom 0.406: Q1.1 19.13,23.69 R13.1 17.72,23.69 19.62,25.59 U2.6
N$46  (via drill 0.35)
  Bottom 0.406: U2.3 24.46,22.42 27.56,22.42 R12A.2 29.21,23.31 R12B.2 v29.21,17.65
VCC  (via drill 0.35)
  Top 0.406: v9.65,27.27 J2.VCC 10.79,27.53 v10.79,28.7 | J1.VCC 5.74,16.61 9.14,13.21 U1.3
  Top 0.61: S1.COMMON 4.38,33.41 SJ2.1@V SJ1.1
  Bottom 0.406: v9.65,27.27 8.89,26.51 8.89,11.56 U1.3 9.6,10.85 9.6,10.82 17.37,3.05 J11.+ | J13.VCC 9.14,30.35 v10.79,28.7 | R9.2 R10.2 C3.1 R11.2 30.42,13.53 31.37,14.48 31.37,17.4 U3.P$8 31.84,19.47 31.84,25.44 30.1,27.18 25.02,27.18 23.11,29.08 23.11,30.35 24.13,31.37
  Bottom 0.61: v9.65,27.27 4.83,32.1 SJ2.1@V 4.83,36.2 6.6,37.97 9.78,37.97 14.22,42.42 | v17.4,45.59 14.22,42.42 | S4.P$5 42.8,34.02 41.5,32.72 41.5,32.1 40.77,31.37 24.13,31.37 22.1,31.37 14.22,39.24 14.22,42.42
  pour Top: 4.22,33.46 4.7,33.93 4.7,32.98
  pour Bottom (no thermals): 14.22,42.42 14.22,39.24 11.05,39.24
  pour Bottom (no thermals): 24.13,31.37 22.1,31.37 23.11,30.35
  pour Bottom (no thermals): 9.65,27.3 8.89,26.54 8.89,28.07

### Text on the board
Bottom: v3.0
tPlace: digitalconcepts.net.au | 8558-BHWSL v3.0
bPlace: S/N | 1 | 2 | 3 | 4
tNames: Vext | Vint | VCC | RAIN | DIR* | SPD | GND | VCC | GND | SCL | SDA | ON
bNames: Vcc | GND | Boost | SDA | SCL | GND | Boost | Bypass | VCC | GPIO38* | GPIO39 | GPIO40 | GPIO45 | GPIO46* | GPIO7 | R12 | GPIO6 | GPIO5 | GPIO4 | GPIO2 | J6A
